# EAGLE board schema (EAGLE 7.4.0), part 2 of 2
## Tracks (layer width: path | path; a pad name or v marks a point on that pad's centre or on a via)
+3V3  (via drill 0.6, 0.8)  (3 unrouted)
  Top 0.254: R29.P$2 183.22,62.91 184.25,63.94 189.55,63.94 189.7,63.79 | IC1.P$64 138.6,54.84 138.8,54.64 139.55,54.64 140,54.19 140,52.23 C11.P$1 | IC1.P$13 142.05,63.44 142.85,64.24 142.85,65.06 C14.P$1 145.3,66.32 C16.P$1 146.5,65.88 146.5,66.41 | IC1.P$19 137.6,68.59 138.2,69.19 138.2,69.78 C12.P$1 | IC1.P$32 131.1,67.41 C15.P$1 | IC1.P$48 129.1,54.59 v128.8,54.29 128.21,54.88 C9.P$1 | IC1.P$64 140.42,55.44 C10.P$1 | IC1.P$64 138.6,56.6 138.95,56.95 | IC1.P$1 139.44,57.44 138.95,56.95 | 138.95,57.06 138.95,56.95
  Top 0.305: IC2.P$3 99.16,24.46 C6.P$1
  Top 0.406: R26.P$2 19.97,60.06 | 23.97,71.79 R27.P$2 | v47.75,104.84 58.65,104.84 60.45,106.64 60.45,107.31 | 143.65,92.19 v143.4,91.94 | v160.5,105.59 160.5,107.26 | v179.93,99.21 184.2,94.94 184.2,80.04 188.5,75.74 R28.P$2 189.28,72.91 190.3,71.89 190.3,67.94 191.7,66.54 | 191.7,66.54 195.38,66.54 R30.P$2 | 191.7,66.54 189.7,64.54 189.7,63.79 | C10.P$1 140.8,55.03 140.8,53.7 141.21,53.3 143.88,53.3 144.03,53.15 144.03,52.96 C13.P$1 | 146.5,66.41 147.38,67.29 151.75,67.29 152.45,66.59 152.45,64.96 151.45,63.84 v151.45,63.64 | v139,71.49 139,70.76 C12.P$1 | v126.65,69.09 128.79,69.09 C15.P$1 | C11.P$1 138.77,49.89 R34.P$2 | 97.21,18.35 IC2.P$15 IC2.P$14 IC2.P$13 95.91,17.5 | 97.21,18.35 97.21,18.5 99.16,20.45 99.16,20.74 | IC2.P$3 99.16,20.74 | C5.P$1 97.72,28.06 99.75,26.04 C6.P$1 | 99.16,20.74 99.31,20.89 100.75,20.89 103.1,23.24 v128.5,23.24 | TP4.TP 78,49.54 76.45,51.09 | U$33.P$4 147.57,21.87 v145,24.44 | 25,46.79 25.78,46.79 25.8,46.81 | 49.67,42.76 49.62,42.76 v44.3,37.44 | v133.2,59.24 133.2,58.29 134.1,57.39 138.62,57.39 138.95,57.06 | v92.75,16.29 93.71,17.25 93.71,18.35 97.21,18.35 | 66,57.29 84.5,57.29 84.5,45.29 66,45.29 66,57.29
  Top 0.813: C2.P$1 49.67,42.76 33.35,26.44 v33.35,12.59 | C5.P$1 93.92,28.06 v91.85,25.99 | v86.4,55.19 77.55,55.19 76.45,54.09 76.45,51.09 76.45,50.99 REG1.P$4 | v135.35,24.09 133.9,24.09 v131.85,22.04 | v44.3,37.44 34.92,46.81 25.8,46.81 25.22,46.81 | 25,46.79 19.97,51.81 R26.P$2 | 19.97,60.06 20.2,60.29 20.2,60.51 21.67,61.99 R33.P$2 22.25,63.06 22.25,70.36 23.55,71.66 R27.P$2 41.75,89.31 v41.75,90.04 | v95.25,76.24 v113.42,76.24
  Top 1.016: C3.P$1 75.45,41.1 REG1.P$2 REG1.P$4 69.42,43.96 C2.P$1
  Bottom 0.406: v143.4,91.94 149.72,91.94 150.25,91.41 152,91.41 157,96.41 157,102.09 v160.5,105.59 166.25,99.84 179.3,99.84 v179.93,99.21 | v151.45,63.64 151.15,63.34 149,63.34 145.7,66.64 145.7,70.89 145.1,71.49 v139,71.49 129.05,71.49 v126.65,69.09 | v128.8,54.29 128.8,55.29 132.35,58.84 | R6.P$2 R5.P$2 91.12,16.29 v92.75,16.29 | SV1.1 33.15,12.39 v33.35,12.59 | 41.85,89.94 v41.75,90.04 41.75,98.84 v47.75,104.84
  Bottom 0.61: v126.65,69.09 126.65,64.34 132.15,58.84 132.35,58.84 132.8,58.84 v133.2,59.24 | C61.P$1 142.98,22.42 v145,24.44
  Bottom 0.813: v91.85,25.99 55.75,25.99 45.26,36.48 | 126.7,69.09 126.7,71.24 135.75,80.29 135.75,83.54 v135.15,84.14 | v86.4,55.19 92.65,61.44 92.65,73.64 v95.25,76.24 | v145,24.44 135.7,24.44 v135.35,24.09 | v131.85,22.04 129.7,22.04 v128.5,23.24 | 45.26,36.48 45.26,36.49 | 45.26,36.48 v44.3,37.44 | v113.42,76.24 121.33,84.14 v135.15,84.14 | v135.15,84.14 135.15,88.49 138.6,91.94 v143.4,91.94
  pour Top (isolate 0.406, no thermals): 84.42,45.34 65.92,45.34 65.92,57.34 84.42,57.34
+5V  (via drill 0.6, 0.8)  (1 unrouted)
  Top 0.254: 150.65,98.51 150.3,98.51 149.94,98.87 IC5.P$1 149.94,108.09 149.82,108.21 149.95,108.21 150.03,108.14 | 150.65,98.51 151.71,98.51 C24.P$1 | IC5.P$7 148.44,96.31 150.65,98.51 | IC6.P$7 177.83,38.65 179.32,37.16 | 179.32,37.16 180.39,37.16 IC6.P$1 180.41,37.16 181.38,37.16 183.28,35.26 195.68,35.26 | C26.P$1 179.27,37.1 179.32,37.16 | IC4.P$7 54.3,96.44 | 54.3,96.44 55.83,97.96 55.83,98.51 | 55.83,98.51 55.83,99.02 IC4.P$1 | C22.P$1 56.49,97.85 55.83,98.51 | R11.P$2 37.4,106.16 41.05,102.51 41.05,101.91 41.67,101.29 43.8,101.29 48.15,96.94 53.81,96.94 54.3,96.44 | IC3.P$1 27.33,36.1 | 27.33,36.1 27.98,36.1 29.38,34.71 | 29.38,34.71 29.48,34.6 IC3.P$7 | C20.P$1 27.37,36.15 27.33,36.1 | 28.95,33.86 28.95,34.29 29.38,34.71 | IC7.5 114.97,12.43 114.51,11.97 112.13,11.97 110.59,13.51 110.59,13.74 110.06,14.27 108.8,14.27 108.5,13.97 108.5,13.94 108.48,13.92 108.46,13.92 108.44,13.9 108.44,13.12 Q1.E
  Top 0.406: v185.93,104.09 185.93,104.06 184.82,104.06 184.3,104.59 184.3,106.51 185.35,107.56 187.75,107.56 R43.P$2 | C25.P$1 153.56,98.08 153,98.64 151.83,98.64 C24.P$1 | R15.P$2 137.53,108.16 137.47,108.21 | v193.4,53.41 196,53.41 | C26.P$1 179.27,32.75 C27.P$1 | T3.P$3 35.46,109.13 | C22.P$1 59.96,97.85 C23.P$1 | R7.P$2 14.7,39.51 14.65,39.56 | C20.P$1 27.37,41.39 C21.P$1 | 15.4,32.86 24.85,32.86 25.28,32.44 27.53,32.44 28.95,33.86 | v16.75,40.64 15.35,40.64 15.25,40.54 | v106,4.66 106,4.48 106.18,4.3 | R19.P$2 199.4,81.39 T7.P$3
  Top 0.813: Q1.E 107.32,9.19 108.99,7.52 LCD.1
  Top 1.016: C4.P$1 77.75,41.57 REG1.P$3 80.64,43.69 C1.P$1 81.8,42.54 84.45,42.54 85.25,41.74 85.25,37.59 70.55,22.89 v69.8,22.89
  Bottom 0.254: C31.P$1 192.56,52.57 v193.4,53.41
  Bottom 0.406: 185.72,103.89 v185.93,104.09 | v193.4,53.41 192.57,52.59 183.85,52.59 182.8,51.54 U$2.P$3 181.12,50.81 R37.P$2 | U$5.P$3 25.03,112.16 | 25.03,112.16 25.92,113.06 33.64,113.06 T3.P$3 | 25.03,112.16 25.02,112.15 23.51,112.15 C43.P$1 | 23.52,111.66 C43.P$1 | 23.3,111.88 C43.P$1 | 11.75,36.84 v11.72,36.86 12.08,36.51 R55.P$2 13.6,35.58 C49.P$1 | C43.P$1 23.2,111.85 23.2,110.31 R49.P$2 21.85,108.96 21.85,109.61 21.17,110.29 20.42,110.29 19.8,110.91 C37.P$1 | U$6.P$3 18.1,39.29 v16.75,40.64 | LCD.1 108.86,7.52 v106,4.66 | 185.8,104.21 v185.93,104.09 | U$4.P$3 185.47,104.54 v185.93,104.09
  Bottom 0.813: R37.P$2 181.03,50.84
  Bottom 1.016: v69.8,22.89 34.38,22.89 30.88,19.39 14.7,19.39
  other vias: 14.72,19.39
  pour Top (isolate 1.016): 2.25,2.29 15.5,2.29 15.5,107.29 195.5,107.29 195.5,2.29 208.75,2.29 208.75,120.54 2.25,120.54
  pour Top (isolate 1.016): 15.5,2.29 195.5,2.29 195.5,22.91 186.75,9.29 15.5,9.29
A12
  Top 0.254: 143.28,60.94 143.88,61.54 146.38,61.54 147,60.91 151.12,60.91 152.5,59.54 154.75,59.54
  Top 0.406: 157.18,59.54 170.5,59.54 173.78,56.26 173.78,53.41 R22.P$2 173.8,51.26 R21.P$1 | 157.18,59.54 154.75,59.54 | C33.P$1 157.6,59.11 157.18,59.54
ADC0
  Top 0.254: IC1.P$14 141.78,63.94 142.25,64.41 142.25,65.29 142.88,65.91 142.88,67.04 143.25,67.41 146.5,67.41 147,67.91 152.72,67.91 154.78,65.86 155.15,65.86
  Top 0.406: R18.P$2 185.07,73.09 R17.P$1 183.22,72.94 183.22,71.81 182.1,70.69 177.55,70.69 172.72,65.86 167.6,65.86 | 167.6,65.86 155.15,65.86 | C39.P$1 167.63,65.83 167.6,65.86
ADC1
  Top 0.254: IC1.P$15 141.53,64.44 141.75,64.66 141.75,65.54 142.38,66.16 142.38,67.29 143,67.91 146.25,67.91 146.75,68.41 153.03,68.41 154.62,66.81 155.15,66.81 | 161.1,66.81 168.57,66.81
  Top 0.406: JP3.1 185.85,66.89 188.5,69.54 R28.P$1 188,71.16 186.88,72.29 186.88,74.54 184.75,76.66 181.75,76.66 171.9,66.81 161.1,66.81 | 161.1,66.81 155.15,66.81 | C57.P$1 161.3,67.01 161.1,66.81
ADC2
  Top 0.254: IC1.P$16 140.6,65.26 141.75,66.41 141.75,67.54 142.62,68.41 146,68.41 146.62,69.04 151.5,69.04 152,69.54
  Top 0.406: 152,72.56 152,86.41 161.12,95.54 169.55,95.54 175.57,101.56 175.57,104.44 R46.P$1 177.5,104.51 R45.P$1 | 152,72.56 152,69.54 | C38.P$1 152,72.56
ADC3  (via drill 0.6)
  Top 0.254: 143.6,69.04 145.75,69.04 146.38,69.66 150.62,69.66 151.12,70.16 | 143.6,69.04 142.38,69.04 141.12,67.79 138.75,67.79 138.6,67.64 IC1.P$17 | C54.P$1 144.25,69.69 143.6,69.04
  Top 0.406: R31.P$1 U$10.2 | v151.12,92.91 151.12,70.16
  Bottom 0.406: U$10.2 156.77,105.56 155.62,104.41 155.62,96.54 152.75,93.66 151.88,93.66 v151.12,92.91
ADC4  (via drill 0.6)  (1 unrouted)
  Top 0.254: IC1.P$20 137.1,76.12 137.25,76.27 137.25,76.79
  Top 0.406: U$12.2 58.67,107.29 R32.P$1 | v64,98.66 117.5,98.66 137.25,78.91 137.25,77.49 | 137.25,77.49 137.25,76.79 | C53.P$1 137.4,77.64 137.25,77.49
  Bottom 0.406: 56.75,107.16 56.75,106.16 57.88,106.16 64,100.04 v64,98.66
ADC5  (via drill 0.6)
  Top 0.254: IC1.P$21 136.6,76.06 136.38,76.29 136.38,76.79
  Top 0.406: 127.08,87.71 117,97.79 72.3,97.79 v70.65,96.14 | 127.08,87.71 136.38,78.41 136.38,76.79 | C44.P$1 126.97,87.61 127.08,87.71 | R51.P$1 R52.P$1 36.62,104.16 v40.25,100.54
  Bottom 0.406: v40.25,100.54 41.38,100.54 49.62,108.79 58,108.79 v70.65,96.14
ADC6
  Top 0.254: IC1.P$22 136.1,75.44 135.5,76.04 135.5,76.79
  Top 0.406: R14.P$2 29.25,71.76 | 29.25,71.76 29.25,72.29 30.12,73.16 35.5,73.16 41.12,67.54 114.5,67.54 117.38,70.41 117.38,75.04 120.88,78.54 126.28,78.54 | 29.25,71.76 R13.P$1 | 126.28,78.54 134.88,78.54 135.5,77.91 135.5,76.79 | C45.P$1 126.12,78.7 126.28,78.54
ADC7
  Top 0.254: IC1.P$23 135.6,75.06 134.62,76.04 134.62,76.79
  Top 0.406: R27.P$1 24.1,67.34 JP2.1 25.15,64.89 26.25,63.79 38.25,63.79 40.25,65.79 | 134.62,76.79 134.62,77.41 134.38,77.66 121.25,77.66 118.25,74.66 118.25,69.91 115,66.66 41.12,66.66 40.25,65.79 | C58.P$1 40.25,65.79
ADC8
  Top 0.254: IC1.P$26 134.1,73.94 133.38,74.66
  Top 0.406: R10.P$2 26.97,52.29 R9.P$1 28.33,52.74 29.38,53.79 33.75,53.79 38.5,58.54 38.5,60.04 | 38.5,60.04 38.5,60.29 42.25,64.04 116.16,64.04 120.88,68.73 120.88,73.41 122.5,75.04 133,75.04 133.38,74.66 | C51.P$1 38.12,59.66 38.5,60.04
ADC9  (via drill 0.6)  (1 unrouted)
  Top 0.254: 133.38,73.66 133.6,73.44 IC1.P$27
  Top 0.406: v22,56.54 22,56.29 25.12,53.16 25.12,51.41 26,50.54 31.88,50.54 39.38,58.04 39.38,59.91 42.62,63.16 101.9,63.16 | 101.9,63.16 116.6,63.16 121.75,68.48 121.75,73.04 122.88,74.16 132.88,74.16 133.38,73.66 | C50.P$1 101.99,63.07 101.9,63.16 | R58.P$1 26.03,43.56 R57.P$1 25.33,43.86 25.33,44.84 18.67,51.49 18.67,54.39 18.65,54.41
  Bottom 0.406: v18.62,54.41 19.88,54.41 v22,56.54
ADC11
  Top 0.254: IC1.P$9 143.03,61.44 143.62,62.04 146.62,62.04 147.25,61.41 151.62,61.41 152.75,60.29 155.25,60.29
  Top 0.406: 154.75,60.29 155.25,60.29 171.12,60.29 177.62,53.79 182.05,53.79 R40.P$1 183.18,52.66 183.18,52.06 184.52,50.72 184.52,50.58 | C28.P$1 184.52,50.58 | 184.52,50.58 R39.P$1
ADC12  (via drill 0.6)
  Top 0.254: IC1.P$10 142.78,61.94 143.38,62.54 146.88,62.54 147.5,61.91 152,61.91 152.88,61.04 154.75,61.04 154.88,61.04
  Top 0.406: 154.75,61.04 180.88,61.04 182.75,59.16 v185.38,59.16 | v191.88,60.04 192.98,60.04 U$9.2 195.5,64.66 R30.P$1
  Bottom 0.406: v191.88,60.04 190.88,61.04 187,61.04 185.38,59.41 v185.38,59.16 184.9,59.64 C55.P$1
ADC13
  Top 0.254: IC1.P$11 142.53,62.44 143.12,63.04 147.12,63.04 147.75,62.41 152.5,62.41 153.12,61.79 154.75,61.79 154.88,61.79
  Top 0.406: 154.75,61.79 181.62,61.79 182.12,61.29 182.75,61.29 R29.P$1 186.5,61.16 187.5,60.16 187.5,58.44 | 187.5,58.44 187.5,57.94 JP4.1 | C56.P$1 188.58,57.35 187.5,58.44
ADC14  (via drill 0.6)
  Top 0.254: IC1.P$24 135.1,74.81 134,75.91 134,76.54 133.75,76.79 133.12,76.79
  Top 0.406: 27.5,61.54 v27.5,61.29 30.38,61.29 32,62.91 38.62,62.91 41.5,65.79 105,65.79 109.1,65.77 115.39,65.77 119.12,69.51 119.12,74.29 121.62,76.79 133.12,76.79 | R33.P$1 19.92,64.21 v20.5,64.79
  Bottom 0.406: U$15.2 17.52,62.56 19.75,64.79 v20.5,64.79 22.62,64.79 24.62,62.79 26,62.79 v27.5,61.29 26.83,60.62 C52.P$1
ADC15
  Top 0.254: IC1.P$25 134.6,74.44 133.38,75.66
  Top 0.406: R26.P$1 21.72,59.71 JP1.1 25.15,57.56 27.5,59.91 30.25,59.91 32.38,62.04 39,62.04 41.88,64.91 115.69,64.91 120,69.16 120,73.91 122,75.91 133.12,75.91 133.38,75.66
  Bottom 0.406: JP1.1 25.15,58.52 C59.P$1
D4  (via drill 0.6)  (2 unrouted)
  Top 0.254: IC1.P$41 123.85,60.94 122.1,59.19 121.35,59.19 118.25,56.09 108.3,56.09
  Top 0.406: 108.3,56.09 107.62,55.41 107.62,50.91 104.88,48.16 99.38,48.16 71.5,20.29 35.79,20.29 35.75,20.32
  Bottom 0.254: 22.55,8.8 22.55,11.32 23.08,11.85 24.51,11.85 28.8,16.14
  Bottom 0.305: SWITCHES.4 22.55,8.8
  Bottom 0.406: 35.85,20.39 32.51,17.09 32.5,17.09 31.55,16.14 28.8,16.14
  other vias: 35.78,20.32
D5  (via drill 0.6)
  Top 0.254: IC1.P$42 124.15,60.44 122.2,58.54 121.5,58.54 118.4,55.44 109.42,55.44
  Top 0.406: 109.42,55.44 108.5,54.51 108.5,50.79 105,47.29 99.75,47.29 71.75,19.29 38.5,19.29 37,17.79 37,15.29 v35.5,13.79
  Bottom 0.406: 26.39,7.54 SWITCHES.6 28.15,9.3 28.15,10.39 27.3,11.24 27.3,12.04 29.65,14.39 34.2,14.39 34.8,13.79 v35.5,13.79
D6  (via drill 0.6)
  Top 0.254: IC1.P$43 124.5,59.94 122.45,57.89 121.7,57.89 118.6,54.79 110.85,54.79
  Top 0.406: 110.85,54.79 109.38,53.31 109.38,50.29 105.38,46.29 100,46.29 72,18.29 41.5,18.29 40.5,17.29 v39.25,17.29
  Bottom 0.406: v39.25,17.29 37.25,15.29 29.25,15.29 24.02,10.06 SWITCHES.3
D7
  Top 0.254: IC1.P$44 124.75,59.44 122.6,57.29 121.95,57.29 118.9,54.24 117.2,54.24 116.1,53.14 116.1,51.09 114.95,49.94 110.28,49.94 109.5,49.16
  Top 0.406: SWITCHES.5 28.27,10.06 29.75,11.54 36.5,11.54 42.25,17.29 72.25,17.29 100.25,45.29 105.62,45.29 109.5,49.16
GND  (via drill 0.6)  (2 unrouted)
  Top 0.254: 57.6,95.89 C22.P$2 | 177.55,35.65 C26.P$2 | 176.8,32.29 176.45,32.29 176.78,32.61 C27.P$2 | IC1.P$60 136.6,56.49 136.85,56.74 | 136.85,56.74 137.9,56.74 138.1,56.54 IC1.P$63 138.1,53.71 C11.P$2 | IC1.P$12 142.3,62.94 143.3,63.94 143.76,63.94 C14.P$2 144.3,64.29 144.65,63.94 144.8,63.94 144.95,63.79 147.5,63.79 148.7,64.99 | C12.P$2 138.86,68.59 138.5,68.59 138.1,68.19 IC1.P$18 138.1,65.44 138.25,65.29 138.8,65.29 v140,66.49 140.05,66.54 | v129.5,66.49 130.4,65.59 131.65,65.59 131.6,65.64 IC1.P$31 131.6,68.94 C15.P$2 | C9.P$2 127.92,57.94 IC1.P$47 130.75,57.94 131.97,56.71 | C18.P$1 146.32,57.91 C19.P$1 148.4,57.44 U$1.GND2 148.63,57.95 149.95,59.27 149.95,59.59 U$1.GND1 | 142.84,55.4 143.54,54.56 146.8,54.55 | 151.68,96.54 C24.P$2 | IC6.P$6 175.95,39.99 176.4,40.44 | IC5.P$6 146.43,95.24 146.4,95.24 145.9,94.74 145.8,94.74 | IC4.P$6 52.25,94.59 52.12,94.46 | IC3.P$6 30.75,32.51 30.8,32.46 | 136.85,56.74 131.97,56.74 131.75,56.96
  Top 0.305: 97.25,23.05 IC2.P$6 97.25,22.97 | 97.25,23.05 97.25,22.66 | 97.25,23.05 97.25,24.58
  Top 0.406: R10.P$1 26.97,53.86 27.69,54.58 JP1.2 | JP1.2 | 27.8,56.19 27.8,54.99 | 31.36,30.43 v32.3,29.49 | 29.47,38.89 C20.P$2 | JP2.2 27.75,66.35 R14.P$1 27.75,70.04 | 151.7,96.47 C24.P$2 152.81,96.5 C25.P$2 154.27,95.04 | R18.P$1 185.1,69.89 183.35,68.14 183.35,66.33 JP3.2 183.31,65.85 181,63.54 177.6,63.54 | 27.75,56.35 JP1.2 | C27.P$2 176.9,32.69 177.35,32.24 | C10.P$2 142.84,55.4 | v94.38,10.29 94.38,12.47 | C8.P$2 100.12,13.17 100,13.17 100,13.79 99.5,13.79 | IC2.P$16 97.86,15.43 99.5,13.79 | 99.5,13.79 94.75,13.79 94.38,13.41 94.38,12.49 C7.P$2 | R4.P$1 103.75,12.54 | 103.75,20.79 v103,21.54 | T13.2 155.09,42.19 v156.1,41.19 | TP3.TP 94.99,49.54 U$11.P$1 | U$33.M2 133.85,12.14 135.5,13.79 139.02,13.79 U$33.WP U$33.GND 141.03,16.07 142.75,17.79 | 142.75,17.79 142.75,19.19 U$33.P$6 142.57,17.97 142.75,17.79 | 142.75,17.79 142.75,17.54 143.25,17.04 149.75,17.04 150,17.29 | 150,17.29 150,19.3 U$33.P$3 150.07,17.36 150,17.29 | U$33.M1 163.82,9.47 | 160.25,13.04 152.75,13.04 150,15.79 150,17.29 | U$33.OPT 152.35,37.44 | 150,17.29 151,17.29 v152.75,15.54 | 152.11,57.52 152.11,57.99 U$1.GND1 | 146.8,54.55 146.8,52.36 C13.P$2 | C16.P$2 149.96,65.57 | 149.96,65.57 150.91,65.57 v151.28,65.94 | C36.P$2 189.11,102.1 R44.P$1 | v182.95,47.41 182.95,44.03 C32.P$2 | C58.P$2 35.58,67.65 34.85,68.39 30.5,68.39 30.3,68.19 30.3,66.36 BAT2.2 | 148.7,64.99 149.38,64.99 149.96,65.57 | IC7.2 114.02,16.73 114.08,16.79 112.14,16.79 C60.P$2 111.07,18.44 v109.5,20.01 | R62.P$2 114.81,21.94 v114.84,21.98 | v192.55,37.44 192.55,39.07 C30.P$2
  Top 0.61: 140.12,69.89 C12.P$2 140.4,70.13 140.4,73.19 v141.05,74.34 | 26.05,69.94 26,69.99 | 53.2,61.04 v53.2,60.04 | 149.11,65.44 C16.P$2 | SWITCHES.1 SWITCHES.2 22.87,5.94 41.2,5.94 43.31,8.05 SV1.5
  Top 0.813: 163.82,9.47 164.12,9.47 164.12,11.91
  Top 1.422: 27.8,56.19 30.23,56.19 BAT1.2
  Bottom 0.254: v129.5,66.49 129.6,66.49 | 133.45,60.49 133.45,60.44 | 140.05,66.54 140.05,66.49 | U$4.P$2 183.05,105.19 183.05,102.74 | U$2.P$2 183.47,50.16 183.82,49.81 183.82,48.29 v182.95,47.41 | 26.12,109.86 25.62,110.36 U$5.P$2 25.55,110.36 26.15,109.76 26.15,108.69 24.85,107.39 23.92,107.39 22.3,105.76
  Bottom 0.305: 95.38,20.79 95.38,20.66 | 102,20.79 102.25,20.79 v103,21.54
  Bottom 0.406: 16.53,60.02 U$15.1 14.67,60.02 13.9,60.79 13.9,63.19 15.7,64.99 16.45,64.99 20.2,68.74 24.75,68.74 v26.05,70.04 | v32.3,29.49 31.9,29.99 30.8,31.09 | 183.25,56.23 JP4.2 | U$3.M4 U$3.M2 102.9,2.52 102.88,2.54 94,2.54 94,2.53 U$3.M1 U$3.M3 U$3.P$5 95.06,7.97 94.38,8.66 | 6.12,70.96 4.95,69.79 | v156.1,41.19 160.4,41.19 160.55,41.04 | U$6.P$2 20.15,38.39 v21.78,36.76
  Bottom 0.61: v53.2,60.04 49.55,63.69 49.55,85.79 48.05,87.29 44.7,87.29 | LED3.C LED4.C LED5.C 71.75,6.36 | 47.83,8.79 SV1.5
  Bottom 0.813: 98,95.79 101,95.79 104.5,92.29 104.5,90.41 105.38,89.54
  Bottom 1.016: v65.45,37.04 65.45,31.49 65.65,31.29 65.65,30.34 65.7,30.29 | 105.38,33.91 105.5,33.91 105.5,27.54
  Bottom 1.422: T4.P$3 70.46,111.4 68.35,113.51
  Bottom 1.676: T2.P$3 11.41,76.25 9.14,73.98 | T6.P$3 169.99,111.25 168.21,113.03
  Bottom 2.184: 97.5,95.66 97.5,89.04 113.62,89.04 113.62,95.79 98,95.79 | 105.38,95.16 105.38,89.54
  Bottom 3.81: B1.P$1 104.5,92.29 B3.P$1 | 9.14,73.98 6.12,70.96 | 68.35,113.51 68.21,113.51 63.43,118.29 | 168.21,113.03 163.76,117.48 163.76,117.97 163.44,118.29 | 37.4,61.24 31.25,61.24 | 173,61.24 179.6,61.24
  Bottom 6.452: 37.4,61.24 44.3,61.24 51.8,53.74 | 65.7,30.29 58.6,30.29 52.25,36.64 52.25,53.29 | 151.5,30.29 152.85,30.29 160.55,37.99 160.55,41.04 160.55,55.69 166.1,61.24 173,61.24
  other vias: 33.8,42.89 154.22,70.01 123.12,54.84 147.4,49.84 143.35,43.74 161.5,54.29 172.5,94.29 163.5,75.29 22.25,80.41 80.75,103.41 111.75,103.91 80.75,79.66 105.88,80.66 45.62,28.16 88.5,17.79 83.38,94.91 147.6,73.14 192.75,101.91 190.75,81.04 50.55,101.61 33.28,59.84 150.18,30.34 136.35,39.46 153,101.29 162.5,98.79 172.5,102.29 136,97.29 187.5,54.29 170.5,43.29 152,54.79 173,32.29 193.5,33.29 20.8,15.99 38.2,53.54 41.75,81.41 55.25,71.41 19.25,101.91 30.25,100.41
  pour Bottom: 103.91,66.04 105.5,64.45 105.5,63.18
  pour Bottom (isolate 0.61): 1,121.79 210,121.79 210,0.79 1,0.79
  pour Top (isolate 1.016): 17.5,11.29 193.5,11.29 193.5,21.29 193.5,105.29 187.5,105.29 17.5,105.29
LCD_DATA1  (via drill 0.6)
  Top 0.254: IC1.P$39 128.2,61.94 127.4,62.74 126.35,62.74 v125.85,62.24
  Top 0.406: v127,25.34 v127,41.24 | v127.15,49.15 127.15,50.39 v128,51.24 | v127,20.89 127,13.21 LCD.12
  Bottom 0.406: v125.85,62.24 125.85,53.39 v128,51.24 | v127,20.89 v127,25.34 | v127,41.24 127.15,41.39 v127.15,49.15
LCD_DATA2  (via drill 0.6)
  Top 0.254: v127.05,61.79 127.4,61.79 127.75,61.44 IC1.P$40
  Top 0.406: v125.2,25.34 126,26.29 126,40.44 125.35,41.09 v125.35,41.24 | v124.95,20.94 126,19.89 126,14.75 LCD.10
  Bottom 0.406: v125.35,41.24 125.35,41.69 126.1,42.44 126.1,49.9 126.37,50.17 128.63,50.17 129.4,50.94 129.4,52.29 127.05,54.64 v127.05,61.79 | v124.95,20.94 125.2,21.19 v125.2,25.34
LCD_DATA3  (via drill 0.6)
  Top 0.254: IC1.P$45 125.35,58.94 124.4,57.99 v124.4,57.69
  Top 0.406: v123.6,21.64 123.6,20.39 125,18.99 125,15.5 122.16,12.66 121.37,12.66 LCD.8 | v124.1,26.39 125,27.34 125,39.89 124.1,40.79 v124.1,41.69
  Bottom 0.406: v124.4,57.69 124.75,57.34 124.75,52.84 125.25,52.34 125.25,42.84 v124.1,41.69 | v123.6,21.64 124.1,22.14 v124.1,26.39
LCD_DATA4  (via drill 0.6)
  Top 0.254: IC1.P$61 137.1,47.64 v137.05,47.59
  Top 0.406: v124,35.99 124,28.29 v122.55,26.84 | v119.95,21.64 116.23,17.92 LCD.6
  Bottom 0.406: 137.05,47.64 v137.05,47.59 137.05,47.29 138.6,45.74 138.6,43.29 138.1,42.79 131.4,42.79 130.7,42.08 130.7,39.89 126.79,35.99 v124,35.99 | v119.95,21.64 121.35,23.04 121.35,25.67 122.52,26.84 v122.55,26.84
LCD_E  (via drill 0.6)
  Top 0.254: IC1.P$4 139.6,58.94 v138.75,59.79
  Top 0.406: v123,24.89 123.85,24.04 127.25,24.04 128,24.79 128,40.14 129.05,41.19 v129.05,41.49 | LCD.7 117.55,8.74 117.55,17.49 v121.9,21.84
  Bottom 0.406: v138.75,59.79 137.85,59.79 136.95,58.89 136.95,55.84 135.75,54.64 135.75,50.44 133.55,48.24 129.55,48.24 128.4,47.09 128.4,42.14 v129.05,41.49 | v121.9,21.84 122.57,22.51 122.57,24.45 v123,24.88 v123,24.89
LCD_RS  (via drill 0.6)
  Top 0.254: IC1.P$62 137.6,48.24 v139.3,46.54
  Top 0.406: LCD.11 128.4,12.07 v128.4,18.94 | v130.9,19.74 130.55,20.09 130.55,30.79 131.82,32.06 v131.82,41.16
  Bottom 0.406: v139.3,46.54 139.3,46.24 139.5,46.04 139.5,42.79 138.55,41.84 132.5,41.84 v131.82,41.16 | v128.4,18.94 129.2,19.74 v130.9,19.74
LCD_RW  (via drill 0.6)
  Top 0.254: IC1.P$3 v138.35,58.44
  Top 0.406: v121.25,19.29 123.4,17.14 v123.4,15.74 | v120.15,24.89 120.15,34.09 v118.3,35.94
  Bottom 0.406: v138.35,58.44 137.85,57.94 137.85,55.39 136.8,54.34 136.8,50.19 139.4,47.59 140.1,47.59 140.4,47.29 140.4,42.34 138.95,40.89 133.05,40.89 133.05,40.84 127,34.79 122.5,34.79 122,35.29 118.95,35.29 v118.3,35.94 | v120.15,24.89 118.75,23.49 118.75,21.04 120.5,19.29 v121.25,19.29 | v123.4,15.74 122.6,14.94 122.6,9.44 121.31,8.15 LCD.9
LED1  (via drill 0.6)
  Top 0.254: IC1.P$51 132.1,54.49 132.07,54.46 132.07,49.34 128.82,46.09 116.3,46.09 102.35,32.14 93.5,32.14 75.62,14.24 v52.75,14.24
  Bottom 0.254: v52.75,14.24 52.7,14.24 R23.P$1
LED2  (via drill 0.6)
  Top 0.254: IC1.P$52 132.6,48.91 129.18,45.49 116.5,45.49 102.6,31.59 93.7,31.59 75.45,13.34 v56.3,13.34
  Bottom 0.254: v56.3,13.34 54.8,13.34 R24.P$1
LED3  (via drill 0.6)
  Top 0.254: v60.4,11.74 74.6,11.74 93.9,31.04 102.85,31.04 116.7,44.89 129.38,44.89 133.1,48.61 IC1.P$53
  Bottom 0.254: v60.4,11.74 60.35,11.79 R25.P$1
N$1  (via drill 0.6)
  Top 0.406: IC2.P$12 95.26,14.9 95.38,14.79 v96.12,14.79
  Bottom 0.406: R1.P$2 100.95,13.49 101.62,14.16 101,14.79 v96.12,14.79
N$2
  Top 0.254: U$1.P$2 150.15,57.59 150.15,57.14 149.16,56.15 145.91,56.15 144.76,57.3 C19.P$2 144.7,57.49 143.5,57.49 141.55,59.44 IC1.P$5
N$3  (via drill 0.6)
  Top 0.406: C8.P$1 98.08,11.95 v99.5,10.41
  Bottom 0.406: R1.P$1 99.5,11.16 v99.5,10.41 99.25,10.28 U$3.P$2
N$4  (via drill 0.6)
  Top 0.406: v97.75,10.41 96.88,10.41 96.38,10.91 96.38,12.47 C7.P$1
  Bottom 0.406: U$3.P$3 98.45,9.72 v97.75,10.41 97.75,11.64 R2.P$1
N$5  (via drill 0.6)
  Top 0.406: v93.5,14.41 93.5,14.66 94.62,15.79 94.62,16.24 IC2.P$11
  Bottom 0.406: R2.P$2 94.47,13.44 v93.5,14.41
N$6
  Top 0.254: U$1.P$4 148.04,60.44 144.64,60.44 144.28,60.11 C18.P$2 143.98,59.04 142.78,59.04 141.88,59.94 IC1.P$6
N$7  (via drill 0.6)  (1 unrouted)
  Top 0.305: 102.12,12.74 102.88,13.66 102.88,18.91 103.06,19.1 v103.06,19.54 | v93.88,19.66 93.88,21.04 94.62,21.79
  Top 0.406: R3.P$1 102.88,10.79 102.12,11.54 102.12,12.74 R4.P$2
  Bottom 0.305: v103.06,19.54 94,19.54 v93.88,19.66
N$8  (via drill 0.6)
  Top 0.406: v101.12,10.04 101.12,9.81 102.1,8.84 R3.P$2
  Bottom 0.406: U$3.P$1 100.05,8.96 v101.12,10.04
N$9  (via drill 0.6)
  Top 0.254: IC6.P$2 179.71,37.65 179.15,38.21 179.15,39.51 179.97,40.34 180.57,40.34
  Top 0.406: R35.P$1 v192.4,68.06 | v191.3,63.16 190.65,62.54 190.65,44.36 187.5,41.19 183.18,41.19 182.3,40.31 180.6,40.31 180.57,40.34
  Bottom 0.406: v192.4,68.06 192.4,64.26 v191.3,63.16
N$10  (via drill 0.6)
  Top 0.305: IC2.P$18 99.17,17.75 99.97,18.55 101.11,18.55 v101.25,18.41 101.23,18.43
  Top 0.406: v91.75,13.91 91.38,13.91 91,14.29 91,16.91 v91.75,17.66
  Bottom 0.305: v91.75,17.66 100.5,17.66 v101.25,18.41
  Bottom 0.406: LED1.C 86.95,6.36 88.12,7.54 88.12,10.91 90.5,13.29 91.12,13.29 v91.75,13.91
N$11  (via drill 0.6)
  Top 0.305: IC2.P$17 98.5,18.29 98.85,18.64 v98.85,18.66
  Bottom 0.406: v98.85,18.66 90.75,18.66 90.12,18.04 90.12,16.54 89.12,15.54 89,15.54 86.62,13.16 82.62,13.16 82,12.54 82,7.96 LED2.C
N$12
  Bottom 0.406: R5.P$1 LED1.A
N$13
  Bottom 0.406: R6.P$1 LED2.A
N$14
  Top 0.406: T7.P$1 195.93,76.25 | 195.93,76.25 195.13,76.25 192.5,73.61 | R19.P$1 194.1,78.94 195.93,77.11 195.93,76.25 | 192.5,73.61 192.5,72.61 R35.P$2 | 192.5,73.61 192.5,76.1 C29.P$1
N$15
  Top 0.406: T1.P$1 14.83,46.33 19.65,41.51 19.65,39.56 R7.P$1 19.58,39.39 19.58,38.69 18.06,37.17 C46.P$1 18.06,35.85 19.67,34.24 22.42,34.24 R53.P$2
N$16
  Top 0.254: IC6.P$3 181.33,38.15 183.68,35.81 186.57,35.81 R36.P$1
N$17
  Top 0.254: IC3.P$3 25.48,35.1 25,35.59 25,36.16 25.85,37.01 25.85,41.29 25.12,42.01 23.28,42.01 19.08,46.21 17,48.29
  Top 0.406: 17,48.29 17.03,72.49 17.05,72.49 17.85,73.29 17.85,73.69 R54.P$1
N$18  (1 unrouted)
  Bottom 0.406: U$6.P$4 18.85,42.21
  Bottom 0.813: 18.85,42.21 18.85,42.24 16.46,44.63
  Bottom 1.016: 16.12,45.66 16.12,47.95 R8.P$1 16.69,48.05 16.92,48.29
  Bottom 1.422: 17.06,48.43 16.92,48.58 | 11.59,78.74 14.69,78.74 | T1.P$2 15.01,43.81
  Bottom 3.81: 14.69,78.74 16.92,76.2 16.95,72.94 10.9,66.89 10.9,54.64 16.92,48.62 16.92,48.58 16.92,48.29 16.92,45.08 16.46,44.63 15.65,43.81 15.01,43.81
N$19  (via drill 0.6)
  Top 0.406: R9.P$2 v31.7,52.29
  Bottom 0.406: 29.6,48.09 29.6,46.55 29.8,46.36 | 32.79,53.34 32.75,53.34 v31.7,52.29 | 20.14,42.96 20.14,41.5 U$6.P$5
  Bottom 0.813: 32.75,53.34 32.77,53.34 BAT1.1 | R8.P$2 20.15,45.78 20.15,42.98 20.14,42.96
  Bottom 1.016: 22.75,48.66 23,48.66 | 23,48.66 23.63,48.66 23.86,48.43 | R8.P$2 22.43,48.09 23,48.66
  Bottom 1.422: 23.86,48.43 24.03,48.26 | BAT1.1 32.77,54 32.79,53.98
  Bottom 2.54: 28.03,45.72 28.03,46.36
  Bottom 3.81: 28.03,46.36 29.8,46.36 32.79,46.36 | U$11.P$2 37.33,46.36 32.79,46.36 | B4.P$2 28.03,35.65 28.03,45.72 25.49,48.26 24.03,48.26 | 32.79,46.36 32.79,53.34
N$20
  Top 0.254: R36.P$2 C30.P$1 199.44,41.23 T8.P$1
N$21  (via drill 0.6)
  Top 0.406: C32.P$1 181.11,46.77 | 181.11,46.77 v181.12,46.79 | 181.11,46.77 R38.P$2
  Bottom 0.406: v181.12,46.79 181.12,48.86 R37.P$1 | 181.25,49.19 R37.P$1 | U$2.P$1 181.57,49.51 R37.P$1
N$22
  Top 0.254: C40.P$1 R11.P$1
  Top 0.406: T3.P$1 40.54,108.68 R11.P$1 | C40.P$1 41.42,105.02 41.42,103.76 R47.P$2
N$23  (via drill 0.6)
  Top 0.406: v184.6,47.16 184.57,47.16 184.57,48.74 R39.P$2
  Bottom 0.406: U$2.P$6 185,47.56 v184.6,47.16
N$24
  Top 0.254: IC4.P$3 54.8,99.79 56.6,101.59 73.6,101.59 R48.P$1
N$25  (1 unrouted)
  Bottom 0.406: 28.41,111.65 27.86,111.65 U$5.P$4
  Bottom 0.813: 38.03,111.22 38,111.22 T3.P$2 | 72.64,107.79 72.96,107.79 72.96,108.79 | 30.84,110.55 29.73,111.66 28.41,111.66 28.41,111.65
  Bottom 1.016: 30.84,110.55 R12.P$1 35.26,106.14 35.26,106.36
  Bottom 1.422: 38.03,111.22 38.03,108.11 | 72.96,111.2 72.96,108.79 72.96,108.27
  Bottom 3.81: 39.78,106.36 42.48,106.36 48.2,112.09 61.95,112.09 67.7,106.34 71.21,106.36 72.64,107.79 | 38.03,108.11 39.78,106.36 | 39.78,106.36 35.26,106.36
N$26  (via drill 0.6)
  Top 0.406: R13.P$2 31.08,70.31 v31.2,70.19
  Bottom 0.406: 28.64,105.4 28.72,105.35 | 32.63,69.69 32.77,69.83 | v31.2,70.19 34.36,70.19 34.38,70.17 | 28.28,110.36 U$5.P$5
  Bottom 0.813: 28.28,110.36 29.28,109.36 29.28,106.31 R12.P$2
  Bottom 1.016: 28.64,105.4 27.95,106.08 28.05,106.14 28.28,106.36 28.83,106.36 R12.P$2 29.26,106.29
  Bottom 1.27: 28.72,105.35 28.36,105
  Bottom 1.676: BAT2.1 32.77,69.83 33.11,70.17 34.38,70.17
  Bottom 3.81: U$18.P$2 34.5,70.29 34.38,70.17 34,70.55 34,84.99 26.7,92.29 B3.P$2 22.67,99.25 28.36,105
N$27  (via drill 0.6)
  Top 0.254: IC1.P$50 131.6,54.29 129.69,52.37 120.44,52.37 103.56,35.5 94.99,35.5 v75.34,15.85
  Bottom 0.254: v75.34,15.85 73.64,15.85 U$34.P$1
N$28
  Top 0.254: IC5.P$2 149.44,102.52 147.88,104.09 R41.P$1
N$29
  Top 0.406: R41.P$2 142.03,102.19 C34.P$1 139.28,102.35 R15.P$1 140.54,105.88 T5.P$1
N$30
  Top 0.406: T6.P$1 175.57,111.21 175.57,106.84 174.95,106.21 169.45,106.21 168.38,105.14 R42.P$2 168.38,101.9 C35.P$1
N$31  (via drill 0.6)
  Top 0.254: v151.85,104.31 166.6,104.31 R42.P$1 | IC5.P$3 148.94,101.32 v147.93,102.34
  Bottom 0.254: v147.93,102.34 147.93,102.89 149.35,104.31 v151.85,104.31
N$32
  Bottom 0.406: U$4.P$4 181.9,104.43 181.38,103.91
  Bottom 1.016: 172.72,106.52 172.13,107.11 | 181.38,103.91 174.75,103.91 171.84,106.82
  Bottom 1.27: 138,107.99 138.04,107.95 | 169.77,106.3 170,106.53 | 169.87,106.53 169.77,106.42 170.05,106.42 R16.P$1
  Bottom 1.422: T6.P$2 173,107.98 | T5.P$2 138,107.99
  Bottom 3.81: 138.04,107.95 138.2,107.95 139.63,106.52 143.1,106.52 143.1,106.49 143.15,106.49 149,112.04 161.45,112.04 167.25,106.54 169.87,106.53 170,106.53 171.54,106.52 171.84,106.82 172.13,107.11 173,107.98
N$33  (via drill 0.6)
  Top 0.406: R17.P$2 181.62,73.81 v182.9,75.09
  Bottom 0.406: 178.26,73.09 178.21,73.14 | v182.9,75.09 178.76,75.09 178.21,75.64 | 179.9,105.19 U$4.P$5
  Bottom 0.813: 179.9,105.19 179.08,106.01 179.08,107.27 179.5,107.69
  Bottom 1.016: 179.5,107.69 179.5,108.33 179.81,108.64
  Bottom 1.27: R16.P$2 177.71,106.52 180.04,108.85
  Bottom 1.422: BAT3.1 178.23,69.99 178.21,70.01
  Bottom 2.54: B1.P$2 189.06,92.13
  Bottom 3.81: 189.06,92.13 189.06,107.26 185.67,110.65 182.02,110.65 180.2,109 180.04,108.85 179.81,108.64 | B1.P$2 188.33,84.9 179.64,76.2 178.21,76.2 | 178.21,76.2 173.65,76.2 U$25.P$2 | 178.21,76.2 178.21,75.64 178.21,73.14 178.21,70.01
N$34  (via drill 0.6)
  Top 0.406: 187.72,106.49 R43.P$1 | C36.P$1 188.05,105.29 | 188.05,105.29 188.05,106.11 R43.P$1 | v185.93,106.06 188,106.06 R43.P$1 | R44.P$2 188.1,105.24 188.05,105.29
  Bottom 0.406: 185.82,106.16 v185.93,106.06 185.7,105.84 U$4.P$1
N$35
  Top 0.254: IC4.P$2 55.3,98.29 54.65,97.64 48.42,97.64 44.1,101.96 R47.P$1
N$36
  Top 0.406: R48.P$2 C41.P$1 75.37,111.07 T4.P$1
N$37  (via drill 0.6)
  Top 0.406: R45.P$2 179.95,104.54 v183.2,107.79
  Bottom 0.406: U$4.P$6 181.9,106.49 v183.2,107.79
N$38
  Bottom 0.406: U$5.P$1 24.3,109.06 22.22,106.99 21,106.99 R50.P$2 | R49.P$1 19.97,107.56 R50.P$2 | C42.P$1 20.73,106.8 R50.P$2
N$41
  Bottom 0.61: LED3.A R23.P$2
N$42
  Bottom 0.61: LED4.A R24.P$2
N$43
  Bottom 0.61: LED5.A R25.P$2
N$44
  Top 0.406: Q1.B 107.32,15.68 R59.P$2
N$45
  Top 0.406: T13.3 158.67,46.12 165.8,38.99 165.8,36.69 167,35.49 167,28.89 171.95,23.94 FAN.2
N$46  (via drill 0.6)
  Top 0.406: v23.92,105.79 23.85,105.71 R51.P$2
  Bottom 0.406: U$5.P$6 27.22,107.99 25.03,105.79 v23.92,105.79
N$47
  Top 0.406: R54.P$2 17.75,77.17 C47.P$1 16.7,77.21 12.58,81.33 T2.P$1
N$48  (1 unrouted)
  Top 0.254: 24.17,34.24 24.55,34.24 25.5,33.29 27.1,33.29 27.67,33.86 27.67,34.96 27.03,35.6 IC3.P$2
N$49
  Bottom 0.406: U$6.P$1 21.88,39.29 23.88,37.29 23.88,35.54 23.1,34.76 17.56,34.76 C48.P$1 15.33,34.7 R56.P$2 15.35,34.79 R55.P$1
N$50  (via drill 0.6)
  Top 0.406: v22.3,44.96 22.47,44.96 R57.P$2
  Bottom 0.406: U$6.P$6 20.8,42.35 22.39,43.94 22.39,44.87 v22.3,44.96
N$51
  Top 0.406: Q1.C 109.52,9.17 110,8.69 115.06,8.69 LCD.5
N$52
  Top 0.406: R60.P$2 110.83,16.06 C60.P$1 113,15.82 IC7.3
N$53  (via drill 0.6)
  Top 0.406: v116.65,20.69 116.65,19.79 R61.P$2 114.97,17.82 IC7.1
  Bottom 0.406: LCD.3 113.69,7.68 114.95,8.94 114.95,10.6 117.24,12.89 117.24,20.1 v116.65,20.69
N$56  (via drill 0.6)
  Top 0.406: R61.P$1 113.06,17.99 R62.P$1 111.67,20.35 v111.6,20.28 | v111.44,14.31 111.9,14.31 IC7.4
  Bottom 0.406: v111.6,20.28 111.6,14.47 v111.44,14.31
N$99  (via drill 0.6)
  Top 0.406: R21.P$2 175.57,48.91 v175.55,48.89
  Bottom 0.406: 178,52.29 177.15,51.44 175.65,51.44 175.55,51.54 | v175.55,48.89 175.55,51.54 | 175.55,51.54 175.5,51.59 | B2.P$2 189.29,30.29 189.29,29.08 | 186.38,50.16 U$2.P$5
  Bottom 0.813: 186.38,50.16 187.18,49.36 R20.P$2
  Bottom 1.016: 187.1,44.56 186.9,44.76 187.25,45.11 187.18,45.18 R20.P$2
  Bottom 1.422: 178.21,52.39 178.21,56.26 BAT4.1
  Bottom 1.93: 167.84,52.39 U$32.P$2
  Bottom 3.81: 187.1,43.66 188.84,41.91 188.84,29.53 189.29,29.08 189.48,28.89 | 187.1,43.66 176.37,43.66 U$32.P$2 178,52.29 178.11,52.29 178.21,52.39 | 187.1,43.66 187.1,44.56
NRST  (via drill 0.6)
  Top 0.254: v141.2,51.24 140.38,50.41 140.38,48.99 R34.P$1 | IC1.P$7 142.65,60.44 v143,60.09
  Top 0.406: SV1.4 40.77,10.36 41.65,11.24 44.7,11.24 49.35,6.59 81.35,6.59 81.8,7.04 93.1,7.04 94.05,7.99 101.75,7.99 102.1,7.64 104.4,7.64 104.95,7.09 107.1,7.09 108.35,5.84 127.35,5.84 129.34,7.61 129.65,7.92 v129.65,33.71 | 142.3,49.49 C17.P$1 142.43,48.86 R34.P$1
  Bottom 0.254: v143,60.09 143,53.04 v141.2,51.24
  Bottom 0.406: 141.15,51.14 141.2,51.14 | 141.2,51.14 141.2,38.54 137.5,34.84 130.78,34.84 v129.65,33.71 | v141.2,51.24 141.2,51.14
PC13  (via drill 0.6)
  Top 0.254: IC1.P$2 142.15,57.94 v144.6,55.49
  Top 0.406: T13.1 152.9,44.21 152.9,49.39 149,53.29 149,53.99 v148.95,54.04
  Bottom 0.406: v148.95,54.04 146.05,54.04 v144.6,55.49
PWM1  (via drill 0.6)
  Top 0.254: IC1.P$37 135.99,62.94 v136.37,62.56 | v129.63,49.6 129.59,49.6 129.56,49.57 129.12,49.57 127.59,48.04 119.19,48.04 v118.12,46.97 v118.12,46.98
  Top 0.406: R59.P$1 v107.28,21.9 v107.29,21.91 | v108.3,24.25 108.3,33.15 117.16,42.01 117.84,42.01 v118.07,41.78
  Bottom 0.254: v136.37,62.56 136.37,62.33 136.28,62.24 136.28,61.71 134.47,59.9 134.47,59.05 130.18,54.76 130.18,50.15 v129.63,49.6 | v118.12,46.97 v118.12,46.98
  Bottom 0.406: v107.29,21.91 107.29,23.24 v108.3,24.25 | v118.07,41.78 118.07,46.92 v118.12,46.97
PWM2  (via drill 0.6)
  Top 0.254: IC1.P$38 134.34,62.44 v136.47,60.31 | v131.19,50.38 131.19,49.59 128.67,47.07 121.16,47.07 v121.1,47.01
  Top 0.406: R60.P$1 109.17,18.19 108.16,19.2 108.16,20.81 v109.17,21.82 | v110.46,24.39 110.36,24.39 109.17,25.58 109.17,32.79 116.79,40.41 118.85,40.41 v120,41.56
  Bottom 0.254: v136.47,60.31 136.47,59.93 131.19,54.65 v131.19,50.38
  Bottom 0.406: v109.17,21.82 109.17,23.1 v110.46,24.39 | v120,41.56 120,41.68 119.08,42.6 119.08,46.09 120.02,47.03 121.08,47.03 v121.1,47.01
RX  (via drill 0.6)
  Top 0.254: IC1.P$58 135.6,45.41 136.97,44.04 v137.55,44.04 | v129.78,44.06 116.83,44.06 TP1.TP 101.6,27.04 v101.6,24.29 | v97.1,20.69 97.3,20.89 98.3,20.89 98.51,21.1 IC2.P$4
  Bottom 0.254: v137.55,44.04 v129.78,44.06 | v101.6,24.29 98,20.69 v97.1,20.69
SPI1_CS  (via drill 0.6)
  Top 0.254: IC1.P$54 133.6,35.99 v137.32,32.26 | v153.85,25.56 155.07,24.34 U$33.P$1 | v147.65,25.59 144.38,28.86 v144.38,32.29
  Top 0.406: 155.25,19.55 U$33.P$1
  Bottom 0.254: v137.32,32.26 143.35,32.26 v144.38,32.29 | v147.65,25.59 147.68,25.56 v153.85,25.56
SPI1_MISO
  Top 0.254: IC1.P$56 134.6,44.31 140.2,38.71 U$33.P$7
SPI1_MOSI
  Top 0.254: IC1.P$57 135.1,44.69 138.32,41.46 145.22,41.46 152.53,34.16 152.53,19.41 U$33.P$2
SPI1_SCK  (via drill 0.6)
  Top 0.254: IC1.P$55 134.1,37.11 v137.45,33.76 | v143.22,33.76 143.22,32.54 142.15,31.46 142.15,23.94 145.1,20.99 145.1,19.4 U$33.P$5
  Bottom 0.254: v137.45,33.76 v143.22,33.76
SPI2_CS1  (via drill 0.6)
  Top 0.254: v87.46,38.76 87.97,39.28 89.46,39.28 92.9,42.71 92.9,42.74 99.14,48.98 104.61,48.98 106.83,51.19 106.83,55.66 107.86,56.7 117.99,56.7 123.47,62.19 v124.2,62.19 | v64.24,38.84 48.52,38.84 v47.44,37.75 | v40.89,37.31 40.85,37.31 38.24,34.7 33.1,34.7 32.2,35.6 IC3.P$9 | IC1.P$33 126.25,64.94 v124.65,66.54
  Bottom 0.254: v87.46,38.76 64.31,38.76 v64.24,38.84 | v47.44,37.75 46.41,37.75 45.25,38.91 42.49,38.91 v40.89,37.31 | v124.65,66.54 124.65,62.64 v124.2,62.19
SPI2_CS2  (via drill 0.6)
  Top 0.254: v116.3,73.75 70.22,73.75 55.31,88.66 55.31,94.58 IC4.P$9 | IC1.P$30 132.1,70.41 131.6,70.91 125,70.91 v123.17,72.74
  Bottom 0.254: v123.17,72.74 117.31,72.74 v116.3,73.75
SPI2_CS3  (via drill 0.6)
  Top 0.254: IC1.P$29 132.6,70.76 v130.51,72.85 | v149.1,90.3 149.44,90.65 IC5.P$9
  Bottom 0.254: v130.51,72.85 130.51,73.43 136.99,79.9 136.99,88.13 139.6,90.74 148.26,90.74 148.7,90.3 v149.1,90.3
SPI2_CS4  (via drill 0.6)  (1 unrouted)
  Top 0.254: IC1.P$28 133.1,72.11 v132.43,72.79 | v156.26,49.2 158.36,49.2 170,37.65 | IC6.P$9 170.01,37.65
  Bottom 0.254: v132.43,72.79 145.34,72.79 147.15,70.98 147.15,67.55 149.57,65.12 149.59,65.12 149.89,64.83 152.6,64.83 153.95,63.48 153.95,51.51 v156.26,49.2
SPI2_MOSI  (via drill 0.6)
  Top 0.254: IC1.P$36 125.45,63.44 | v37.1,33.54 33.3,33.54 31.75,35.09 30.76,35.09 IC3.P$8 | v60.25,76.29 60.25,82.74 54.8,88.18 IC4.P$8 | IC6.P$8 170.28,38.15 157.6,50.84 157.6,52.09 v156.35,53.34 | IC5.P$8 148.94,91.68 146.3,89.04 146.3,86.94 v146.4,86.84
  Top 0.406: 125.45,63.44 123.15,63.44 117.8,58.09 96.5,58.09 96.15,58.44 61.2,58.44 | v45.65,44.34 59.75,58.44 61.2,58.44 | 61.2,58.44 v62.1,57.54 | v146.4,86.84 136.8,86.84 134.85,88.79 131.4,88.79 130.3,87.69 130.3,87.24 131.8,85.74 133,85.74 v133.25,85.99 | v118.1,84.74 118.1,85.44 117.1,86.44 95.15,86.44 v93.6,84.89
  Bottom 0.406: v45.65,44.34 45.6,44.34 38.9,37.64 38.9,35.34 v37.1,33.54 | v62.1,57.54 62.1,69.04 62.85,69.79 62.85,70.94 61.9,71.89 61.9,74.64 v60.25,76.29 88.6,76.29 93.6,81.29 v93.6,84.89 | v156.35,53.34 156.35,54.59 155.5,55.44 155.5,66.79 151.65,70.64 151.65,83.24 148.05,86.84 v146.4,86.84 | v133.25,85.99 119.35,85.99 v118.1,84.74
SPI2_SCK  (via drill 0.6)
  Top 0.254: IC3.P$10 32.46,36.1 33.35,35.21 36.06,35.21 37.26,36.41 | IC1.P$34 125.45,64.44 | IC4.P$10 55.8,88.93 60.7,84.04 v61.4,84.04 | IC6.P$10 169.58,37.15 159.15,47.59 156.35,47.59 154.65,49.29 154.65,50.59 v155.6,51.54 | IC5.P$10 149.94,91.19 150.3,90.84 150.3,87.79 v147.95,85.44
  Top 0.406: 125.45,64.44 122.9,64.44 117.45,58.99 97.25,58.99 96.75,59.49 58.65,59.49 | v39.15,40.04 39.15,38.3 37.26,36.41 | 58.65,59.49 v42.75,43.59 | 58.65,59.49 v55.85,59.49 | v61.4,70.34 v61.4,78.84 | v147.95,85.44 136.65,85.44 134.55,87.54 v131.9,87.54 | v118.25,87.49 93.65,87.49 v93.6,87.54
  Bottom 0.406: v42.75,43.59 42.7,43.59 v39.15,40.04 | v55.85,59.49 55.85,64.79 v61.4,70.34 | v61.4,78.84 v61.4,84.04 64.9,87.54 v93.6,87.54 | v147.95,85.44 150.5,82.89 150.5,70.39 154.65,66.24 154.65,52.49 v155.6,51.54 | v131.9,87.54 118.3,87.54 v118.25,87.49
SWCLK
  Top 0.254: IC1.P$49 131.1,54.84 129.3,53.04 117.65,53.04 117.35,52.74 117.35,50.64 115.55,48.84 111.5,48.84
  Top 0.406: SV1.3 38.23,10.52 43.25,15.54 72.75,15.54 100.5,43.29 105.95,43.29 111.5,48.84
SWDIO
  Top 0.254: IC1.P$46 127.6,58.44 125.9,56.74 122.2,56.74 119.1,53.64 117.4,53.64 116.7,52.94 116.7,50.89 115.2,49.39 110.85,49.39 110.5,49.04
  Top 0.406: SV1.2 35.69,9.23 42.88,16.41 72.5,16.41 100.38,44.29 105.75,44.29 110.5,49.04
T
  Bottom 0.406: U$2.P$4 185.03,50.81 185.7,51.49 186.75,51.49 186.78,51.46
  Bottom 0.813: 193.12,47.21 191.15,49.19 191.15,49.21 188.9,51.46 186.78,51.46 186.24,51.46
  Bottom 1.016: 192.88,47.79 192.88,46.73 | R20.P$1 192.88,46.66 192.88,46.73 | 192.88,46.73 192.81,46.79
  Bottom 1.27: 192.64,47.16 192.81,46.99
  Bottom 1.422: T8.P$2 195.54,43.79
  Bottom 1.676: T7.P$2 196.31,78.79 195.4,78.79 195.35,78.74 | 195.54,43.79 195.51,43.81
  Bottom 3.81: 195.51,43.81 194.24,43.81 192.81,45.24 192.81,46.79 192.81,46.99 192.85,46.94 193.12,47.21 200.05,54.14 200.05,66.04 194.9,71.19 194.9,71.29 192.81,73.37 192.81,75.3 196.31,78.79
TX  (via drill 0.6)
  Top 0.254: IC1.P$59 136.1,46.84 v137.05,45.89 | v132,45.89 132,44.14 130.8,42.94 116.88,42.94 106.2,32.26 106.2,28.04 TP2.TP 106.22,27.81 v106.22,24.46
  Top 0.305: IC2.P$20 100.96,17 v101.65,16.31
  Bottom 0.254: v137.05,45.89 v132,45.89 | v101.65,16.31 102.4,16.31 106.15,20.06 106.15,24.39 v106.22,24.46

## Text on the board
bStop: battery measurement tool / designed by jurajh, ver 1.1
